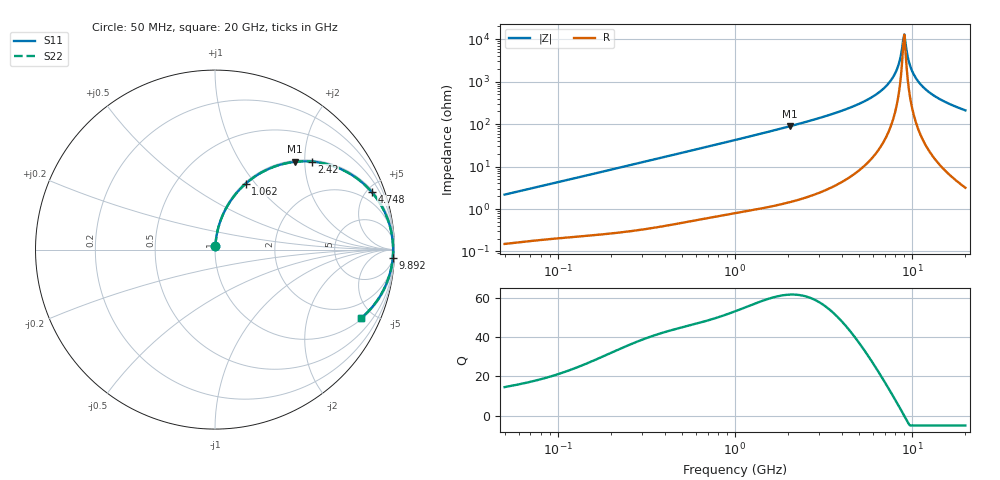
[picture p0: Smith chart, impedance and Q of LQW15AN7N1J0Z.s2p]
!Murata Part Number: LQW15AN7N1J0Z
!These Parameters are Measured in Series Mode Connection
!  o--[Z]--o
!Port1  Port2
!  o-------o
!Freq. Start=50[MHz] Stop=20[GHz], 401[Steps]
# Hz S RI R 50
!Freq.(Hz) S11(Real) S11(Imag) S21(Real) S21(Imag) S12(Real) S12(Imag) S22(Real) S22(Imag)
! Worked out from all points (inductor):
!   401 points, 50 MHz to 20 GHz, reference 50 ohm
!   read as one part in series: L = 6.89 nH near 51.52 MHz
!   highest Q = 61.5 at 2.052 GHz (marker M1), where L = 6.96 nH
!   self-resonance near 8.907 GHz
!   S11 on the Smith chart (normalised r, x): 50 MHz: 1.00, +0.04; 1.062 GHz: 1.02, +0.90; 2.42 GHz: 1.04, +2.16; 4.748 GHz: 1.14, +5.43; 9.892 GHz: 7, -40; 20 GHz: 1.06, -4.22
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5e7  0.00197 0.0217  0.998 -0.0217  0.998 -0.0217  0.00197 0.0217
1.364002e8  0.00562 0.0576  0.9944 -0.0576  0.9944 -0.0576  0.00562 0.0576
3.721004e8  0.0275 0.1521  0.9725 -0.1521  0.9725 -0.1521  0.0275 0.1521
1e9  0.1557 0.3533  0.8443 -0.3533  0.8443 -0.3533  0.1557 0.3533
1.061746e9  0.1719 0.3681  0.8281 -0.3681  0.8281 -0.3681  0.1719 0.3681
2.05233e9  0.4467 0.4891  0.5533 -0.4891  0.5533 -0.4891  0.4467 0.4891
2.419936e9  0.5378 0.4904  0.4622 -0.4904  0.4622 -0.4904  0.5378 0.4904
2.728004e9  0.6054 0.4804  0.3946 -0.4804  0.3946 -0.4804  0.6054 0.4804
4.748272e9  0.8745 0.3189  0.1255 -0.3189  0.1255 -0.3189  0.8745 0.3189
6.217679e9  0.9527 0.1929  0.0473 -0.1929  0.0473 -0.1929  0.9527 0.1929
7.442007e9  0.9817 0.1011  0.0183 -0.1011  0.0183 -0.1011  0.9817 0.1011
8.264682e9  0.9902 0.0462  0.00984 -0.0462  0.00984 -0.0462  0.9902 0.0462
8.516016e9  0.9914 0.0304  0.00857 -0.0304  0.00857 -0.0304  0.9914 0.0304
8.774992e9  0.9922 0.0146  0.00781 -0.0146  0.00781 -0.0146  0.9922 0.0146
9.041845e9  0.9924 -0.0012  0.00756 0.0012  0.00756 0.0012  0.9924 -0.0012
9.178299e9  0.9924 -0.00911  0.00763 0.00911  0.00763 0.00911  0.9924 -0.00911
9.600142e9  0.9914 -0.0328  0.00858 0.0328  0.00858 0.0328  0.9914 -0.0328
9.892087e9  0.9902 -0.0486  0.00985 0.0486  0.00985 0.0486  0.9902 -0.0486
1.082228e10  0.9833 -0.0958  0.0167 0.0958  0.0167 0.0958  0.9833 -0.0958
1.257102e10  0.9616 -0.173  0.0384 0.173  0.0384 0.173  0.9616 -0.173
1.550395e10  0.9096 -0.2752  0.0904 0.2752  0.0904 0.2752  0.9096 -0.2752
2e10  0.8132 -0.3823  0.1868 0.3823  0.1868 0.3823  0.8132 -0.3823
